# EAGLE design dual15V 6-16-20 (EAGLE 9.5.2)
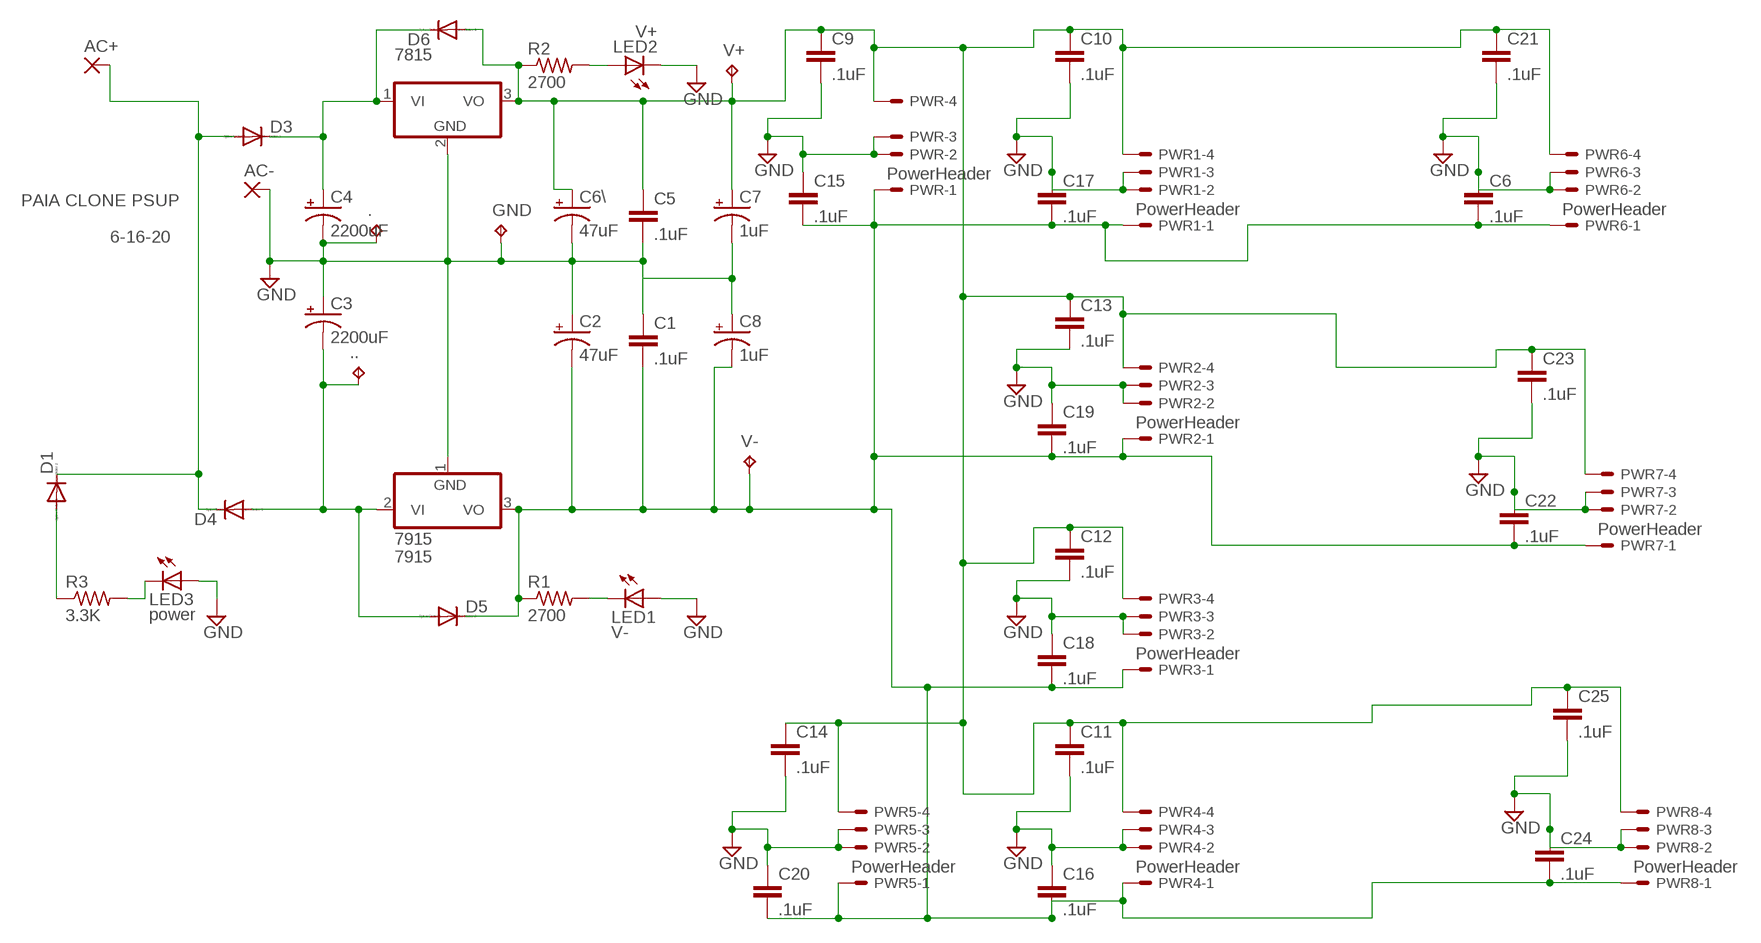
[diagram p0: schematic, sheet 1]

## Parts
7815  7805T  [TO220H]
7915  7915  7905T  [TO220H]
.  TPPAD1-17Y  [P1-17Y]
..  TPPAD1-17Y  [P1-17Y]
AC+  3,17/1,3  [3,17/1,3]
AC-  3,17/1,3  [3,17/1,3]
C1  .1uF  C5/2.5  [C5B2.5]
C2  47uF  CPOL-USE5-8.5  [E5-8,5]
C3  2200uF  CPOL-USE25-10AXIAL  [E25-10]
C4  2200uF  CPOL-USE25-10AXIAL  [E25-10]
C5  .1uF  C5/2.5  [C5B2.5]
C6  .1uF  C2.5/2  [C2.5-2]
C6\  47uF  CPOL-USE5-8.5  [E5-8,5]
C7  1uF  CPOL-USE5-8.5  [E5-8,5]
C8  1uF  CPOL-USE5-8.5  [E5-8,5]
C9  .1uF  C2.5/2  [C2.5-2]
C10  .1uF  C2.5/2  [C2.5-2]
C11  .1uF  C2.5/2  [C2.5-2]
C12  .1uF  C2.5/2  [C2.5-2]
C13  .1uF  C2.5/2  [C2.5-2]
C14  .1uF  C2.5/2  [C2.5-2]
C15  .1uF  C2.5/2  [C2.5-2]
C16  .1uF  C2.5/2  [C2.5-2]
C17  .1uF  C2.5/2  [C2.5-2]
C18  .1uF  C2.5/2  [C2.5-2]
C19  .1uF  C2.5/2  [C2.5-2]
C20  .1uF  C2.5/2  [C2.5-2]
C21  .1uF  C2.5/2  [C2.5-2]
C22  .1uF  C2.5/2  [C2.5-2]
C23  .1uF  C2.5/2  [C2.5-2]
C24  .1uF  C2.5/2  [C2.5-2]
C25  .1uF  C2.5/2  [C2.5-2]
D1  1N4004  [DO41-10]
D3  1N4004  [DO41-10]
D4  1N4004  [DO41-10]
D5  1N4004  [DO41-10]
D6  1N4004  [DO41-10]
GND  TPPAD1-17Y  [P1-17Y]
LED1  V-  LEDB156  [Q62902-B156]
LED2  V+  LEDB156  [Q62902-B156]
LED3  power  LEDB156  [Q62902-B156]
PWR  PowerHeader  C-GRID-04-70543  [70543-04]
PWR1  PowerHeader  C-GRID-04-70543  [70543-04]
PWR2  PowerHeader  C-GRID-04-70543  [70543-04]
PWR3  PowerHeader  C-GRID-04-70543  [70543-04]
PWR4  PowerHeader  C-GRID-04-70543  [70543-04]
PWR5  PowerHeader  C-GRID-04-70543  [70543-04]
PWR6  PowerHeader  C-GRID-04-70543  [70543-04]
PWR7  PowerHeader  C-GRID-04-70543  [70543-04]
PWR8  PowerHeader  C-GRID-04-70543  [70543-04]
R1  2700  R-US_0204/7  [0204/7]
R2  2700  R-US_0204/7  [0204/7]
R3  3.3K  R-US_0204/7  [0204/7]
V+  TPPAD1-17Y  [P1-17Y]
V-  TPPAD1-17Y  [P1-17Y]

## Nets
GND: 7815.2(GND) 7915.1(GND) ..TP AC-.1(P) C1.1 C2.+ C3.+ C4.- C5.2 C6.1 C6\.- C7.- C8.+ C9.2 C10.2 C11.2 C12.2 C13.2 C14.2 C15.1 C16.1 C17.1 C18.1 C19.1 C20.1 C21.2 C22.1 C23.2 C24.1 C25.2 GND.TP LED1.A LED2.K(C) LED3.A PWR1.2 PWR1.3 PWR2.2 PWR2.3 PWR3.2 PWR3.3 PWR4.2 PWR4.3 PWR5.2 PWR5.3 PWR6.2 PWR6.3 PWR7.2 PWR7.3 PWR8.2 PWR8.3 PWR.2 PWR.3
N$1: 7815.1(VI) C4.+ D3.C D6.C
N$2: AC+.1(P) D1.C D3.A D4.C
N$3: LED3.K(C) R3.2
N$4: D1.A R3.1
N$5: LED2.A R2.2
N$6: 7915.2(VI) ...TP C3.- D4.A D5.A
N$7: LED1.K(C) R1.2
V+15: 7815.3(VO) C5.1 C6\.+ C7.+ C9.1 C10.1 C11.1 C12.1 C13.1 C14.1 C21.1 C23.1 C25.1 D6.A PWR1.4 PWR2.4 PWR3.4 PWR4.4 PWR5.4 PWR6.4 PWR7.4 PWR8.4 PWR.4 R2.1 V+.TP
V-15: 7915.3(VO) C1.2 C2.- C6.2 C8.- C15.2 C16.2 C17.2 C18.2 C19.2 C20.2 C22.2 C24.2 D5.C PWR1.1 PWR2.1 PWR3.1 PWR4.1 PWR5.1 PWR6.1 PWR7.1 PWR8.1 PWR.1 R1.1 V-.TP

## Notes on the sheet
- PAIA CLONE PSUP
- 6-16-20

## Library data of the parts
7815 = linear:78*: Positive VOLTAGE REGULATOR Source: http://cache.national.com/ds/LM/LM78L05.pdf http://www.fairchildsemi.com/ds/LM/LM7805.pdf
7915 = linear:79*: Negative VOLTAGE REGULATOR
. .. GND V+ V- = testpad:TP: Test pad
AC+ AC- = wirepad:3,17/1,3: THROUGH-HOLE PAD
C1 C5 C6 C9-C25 = capacitor-wima:C: CAPACITOR
C2-C4 C6\ C7 C8 = rcl:CPOL-US: POLARIZED CAPACITOR, American symbol; SPICEPREFIX: C
D1 D3-D6 = diode:1N4004: DIODE
LED1-LED3 = led:LED: LED
PWR PWR1-PWR8 = con-molex:C-GRID-04: CONNECTOR wire to board 2.54 mm (0.100") pitch header; MF: MOLEX; OC_FARNELL: unknown; OC_NEWARK: unknown
R1-R3 = rcl:R-US_: RESISTOR, American symbol

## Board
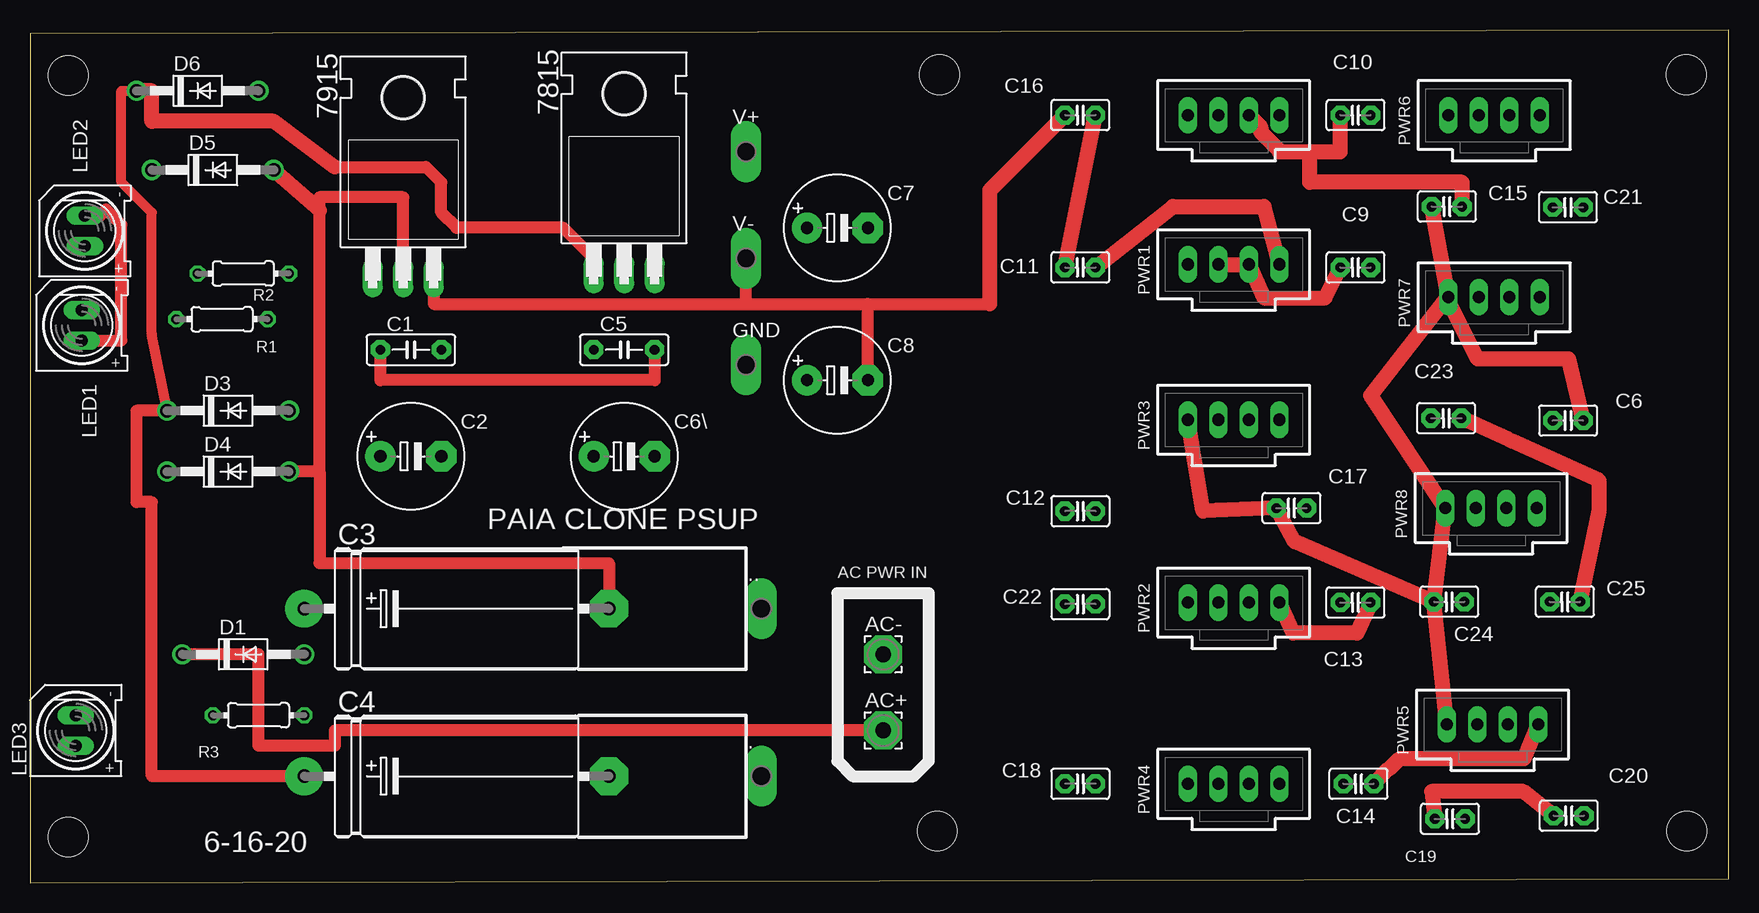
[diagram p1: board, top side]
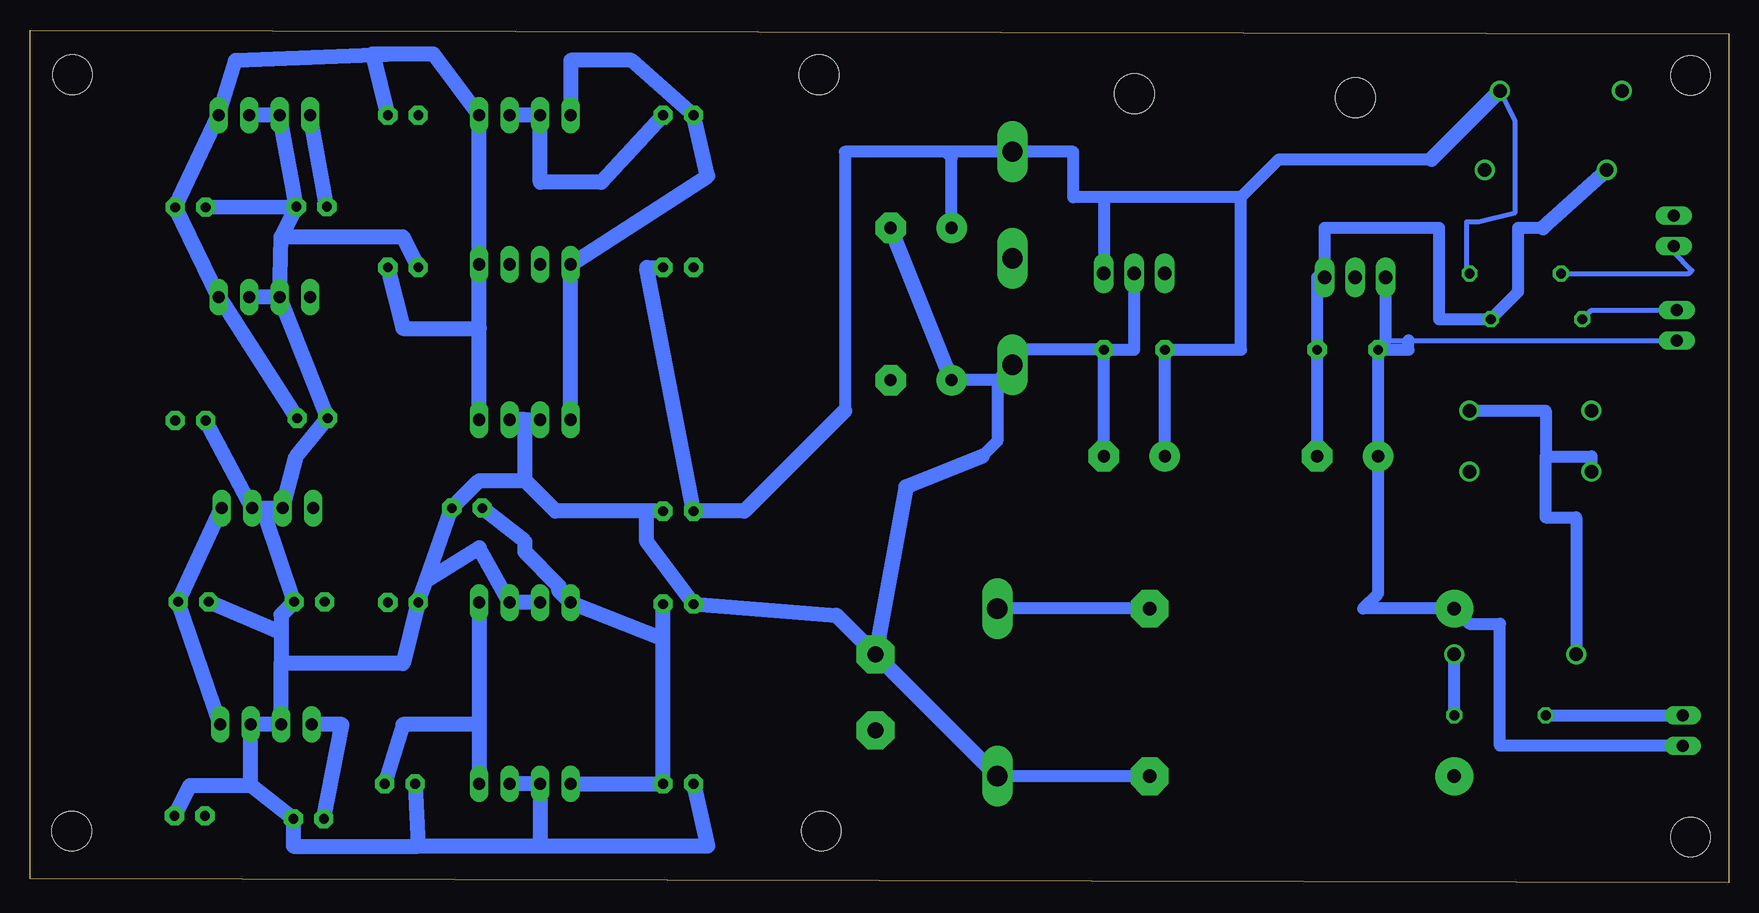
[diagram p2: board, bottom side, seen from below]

Size 141.59 x 71.11 mm. Coordinates in mm from the lower left corner, seen from the top.
Outline: 0,0 141.59,0.32 141.59,71.11 0,70.79 0,0
Copper layers (1*16): Top 0.035mm / dielectric 1.5mm / Bottom 0.035mm
Design rules "default": minimum track width 6mil, minimum drill 0.35mm, track to track 6mil, track to pad 6mil, pad to pad 6mil, via to via 6mil, smd to smd 6mil, copper to edge 40mil, drill to drill 6mil, minimum pad ring 10mil, minimum via ring 8mil, stop-mask expansion 4mil, vias tented up to drill 0mil, thermal gap 10mil
Holes 3.3 mm at 3.17,3.81 75.63,4.32 75.82,67.37 3.17,67.31 138.05,67.37 138.11,4.32

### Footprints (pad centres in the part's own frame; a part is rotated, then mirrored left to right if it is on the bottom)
TO220H = drill 1.118 long: 1 -2.54,-10.16; 2 0,-10.16; 3 2.54,-10.16 | hole 3.302: 0,4.826
P1-17Y = drill 1.702 pad 2.121 long: TP 0,0
3,17/1,3 = drill 1.321 pad 3.175 octagon: 1 0,0
C5B2.5 = drill 0.813 pad 1.6 octagon: 1 -2.54,0; 2 2.54,0
E5-8,5 = drill 1.016 pad 2.54: + -2.54,0 | drill 1.016 pad 2.54 octagon: - 2.54,0
E25-10 = drill 1.118 pad 3.15: + -12.7,0 | drill 1.118 pad 3.15 octagon: - 12.7,0
C2.5-2 = drill 0.813 pad 1.6 octagon: 1 -1.27,0; 2 1.27,0
DO41-10 = drill 1.118: A 5.08,0; C -5.08,0
Q62902-B156 = drill 1.016 long: A -1.27,0; K 1.27,0
70543-04 = drill 1.016 long: 1 -3.81,0; 2 -1.27,0; 3 1.27,0; 4 3.81,0
0204/7 = drill 0.813 octagon: 1 -3.81,0; 2 3.81,0

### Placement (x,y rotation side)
7815  49.53,60.96 0 top
7915  31.11,60.64 0 top
.  60.96,8.89 0 top
..  60.96,22.86 0 top
AC+  71.12,12.7 0 top
AC-  71.12,19.05 0 top
C1  31.75,44.45 0 top
C2  31.75,35.56 0 top
C3  35.56,22.86 0 top
C4  35.56,8.89 0 top
C5  49.53,44.45 0 top
C6  128.21,38.54 0 top
C6\  49.53,35.56 0 top
C7  67.31,54.61 0 top
C8  67.31,41.91 0 top
C9  110.49,51.31 180 top
C10  110.49,64.01 180 top
C11  87.55,51.31 180 top
C12  87.55,30.99 0 top
C13  110.49,23.37 180 top
C14  110.74,8.25 180 top
C15  118.11,56.39 180 top
C16  87.55,64.01 180 top
C17  105.16,31.24 180 top
C18  87.55,8.25 0 top
C19  118.36,5.33 180 top
C20  128.27,5.59 180 top
C21  128.21,56.32 180 top
C22  87.55,23.24 0 top
C23  118.05,38.73 180 top
C24  118.3,23.43 180 top
C25  127.95,23.43 180 top
D1  17.78,19.05 0 top
D3  16.51,39.37 0 top
D4  16.51,34.29 0 top
D5  15.24,59.44 0 top
D6  13.97,66.04 0 top
GND  59.69,43.18 0 top
LED1  4.32,46.48 90 top
LED2  4.57,54.36 90 top
LED3  3.81,12.7 90 top
PWR  100.33,64.01 0 top
PWR1  100.33,51.56 0 top
PWR2  100.33,23.37 0 top
PWR3  100.33,38.61 0 top
PWR4  100.33,8.25 0 top
PWR5  121.92,13.21 0 top
PWR6  122.05,64.01 0 top
PWR7  122.05,48.83 0 top
PWR8  121.79,31.24 0 top
R1  16,46.99 180 top
R2  17.78,50.8 180 top
R3  19.05,13.97 180 top
V+  59.69,60.96 0 top
V-  59.69,52.07 0 top

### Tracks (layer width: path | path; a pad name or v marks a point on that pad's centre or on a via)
GND
  Top 1.016: C5.2 52.07,41.91 29.21,41.91 C1.1 | LED1.A 7.62,45.21 7.62,54.86 6.35,56.13 5.84,55.63 LED2.K
  Top 1.27: C11.2 C16.1 | PWR1.2 PWR1.3 102.87,48.77 107.95,48.77 C9.2 | PWR.3 102.59,63.02 102.59,62.6 104.14,61.06 104.14,60.96 106.68,60.96 | 106.68,60.96 109.22,60.96 C10.2 | C15.1 119.38,58.42 106.68,58.42 106.68,60.96
  Bottom 0.406: 28.57,45.21 26.67,45.21 LED1.A
  Bottom 1.016: C5.2 49.53,44.45 7815.2 | C5.2 59.69,44.45 GND.TP 60.96,41.91 | C6\.- C5.2 | C4.- ..TP | 28.57,45.21 7915.1 | 60.96,41.91 60.96,36.83 62.23,35.56 | 60.96,41.91 C8.+ | LED3.A 19.05,11.43 19.05,21.59 21.59,21.59 C3.+ 30.48,22.86 29.21,24.13 C2.+ C1.1 26.67,44.45 26.67,45.21
  Bottom 1.27: PWR2.2 PWR2.3 104.14,27.94 108.58,25.17 | C12.2 90.17,30.99 | 90.17,30.99 97.79,30.99 100.33,33.53 | 100.33,33.53 100.33,38.61 | 100.33,38.61 PWR3.2 | 100.33,38.61 PWR3.3 | 100.33,33.53 104.14,33.53 C17.1 108.58,25.17 | 90.17,30.99 90.17,28.45 C22.1 74.38,22.31 AC-.1 | 120.65,18.29 110.49,18.29 C13.2 108.58,25.17 | 120.65,20.83 120.65,22.35 C24.1 121.92,30.48 PWR8.3 | 120.65,20.83 120.65,18.29 | 62.23,35.56 68.58,33.02 AC-.1 | ..TP AC-.1 | C15.1 119.74,58.35 PWR6.2 PWR6.3 | PWR7.2 C23.2 119.38,35.56 PWR8.2 PWR8.3 | C18.1 85.09,3.05 99.06,3.05 | 99.06,3.05 109.22,3.05 | 109.22,3.05 119.63,3.05 C19.1 123.19,8.13 | C9.2 110.49,53.85 120.65,53.85 | 120.65,53.85 C15.1 | C21.2 C15.1 | PWR7.2 120.65,53.85 | PWR7.2 PWR7.3 | 120.65,18.29 PWR5.2 PWR5.3 123.19,8.13 | C20.1 128.27,8.13 123.19,8.13 | 120.65,20.83 C25.2 | C8.+ C7.- | C16.1 93.98,58.42 99.06,58.42 PWR.2 PWR.3 | PWR8.3 C6.1 | C14.2 109.22,3.05 | PWR4.3 PWR4.2 99.06,3.05
N$1
  Top 0.813: D3.C 10.16,45.72 10.16,55.88 7.62,58.42 7.62,66.04 D6.C
  Top 1.016: C4.+ 10.16,8.89 10.16,31.75 8.89,31.75 8.89,39.37 D3.C | 7815.1 46.99,52.07 44.45,54.61 35.56,54.61 34.29,55.88 34.29,58.42 33.02,59.69 25.4,59.69
  Top 1.27: 25.4,59.69 20.32,63.5 10.16,63.5 10.16,66.04 D6.C
N$2
  Top 1.016: D1.C 19.05,19.05 19.05,11.43 25.4,11.43 25.4,12.7 AC+.1
  Bottom 1.016: D3.A 15.24,39.37 15.24,35.56 | 15.24,35.56 11.43,35.56 D4.C | 15.24,35.56 15.24,30.48 12.7,30.48 D1.C
N$3
  Bottom 1.016: R3.2 LED3.K
N$4
  Bottom 1.016: R3.1 D1.A
N$5
  Bottom 0.406: R2.2 3.3,50.8 3.05,51.05 4.57,52.58 LED2.A
N$6
  Top 1.016: 7915.2 31.11,57.15 24.13,57.15 24.13,56.07 24.13,34.29 | 24.13,34.29 D4.A | 24.13,34.29 24.13,26.67 48.26,26.67 C3.-
  Top 1.27: D5.A 24.13,56.07
  Bottom 1.016: C3.- ...TP
N$7
  Bottom 0.406: LED1.K 11.43,47.75 R1.2
V+15
  Top 1.27: C11.1 95.25,56.39 102.87,56.39 PWR1.4 | C25.1 130.81,30.99 130.81,33.53 123.53,36.83 123.27,36.94 C23.1 | C13.1 110.61,20.83 105.3,20.83 PWR2.4 | C14.1 113.28,9.53 113.35,9.53 114.19,10.37 124.55,10.37 PWR5.4
  Bottom 0.406: R2.1 21.84,51.05 21.84,55.12 20.83,55.12 17.78,55.88 17.78,63.5 D6.A
  Bottom 1.016: 73.66,39.37 73.66,60.96 65.28,60.96 | C6\.+ C5.1 40.64,44.45 40.64,57.15 | 40.64,57.15 52.07,57.15 | 52.07,57.15 7815.3 | 52.07,57.15 54.61,57.15 54.61,60.96 V+.TP 65.28,60.96 | 24.77,60.33 37.47,60.33 40.64,57.15 | C7.+ 64.77,60.45 65.28,60.96
  Bottom 1.27: 73.66,39.37 82.04,30.99 C12.1 90.17,51.31 C11.1 | PWR2.4 104.14,13.21 | 104.14,13.21 PWR4.4 | 111.76,69.09 107.95,69.09 PWR.4 PWR1.4 104.14,46.23 | 111.76,69.09 113.03,69.09 C10.1 | 104.14,13.21 110.49,13.21 C14.1 | PWR3.4 104.14,46.23 | C9.1 110.49,46.23 104.14,46.23 | C23.1 125.73,48.77 PWR7.4 C21.1 PWR6.4 124.46,68.58 111.76,69.09 | PWR5.4 C25.1 PWR8.4 | 24.77,60.33 D6.A
V-15
  Top 1.016: 7915.3 33.66,48.26 59.69,48.26 | 59.69,48.26 V-.TP | 59.69,48.26 69.85,48.26 | 69.85,48.26 80.01,48.26 | C8.- 69.85,48.26
  Top 1.27: C16.2 80.01,57.74 80.01,48.26 | C15.2 PWR7.1 118.11,48.77 | C6.2 128.27,43.69 120.65,43.69 118.11,48.77 | PWR3.1 97.79,30.99 C17.2 105.41,28.45 C24.2 | PWR5.1 C24.2 | C20.2 124.46,7.62 116.84,7.62 C19.2 | C24.2 PWR8.1 111.76,40.64 118.11,48.77
  Bottom 1.016: C2.- C1.2 34.29,50.48 7915.3 33.66,54.61 24.13,54.61 24.13,46.99 R1.1 17.53,49.28 17.53,54.61 15.47,54.61
  Bottom 1.27: C17.2 100.33,28.45 100.33,27.59 97.51,24.77 97.51,24.36 PWR2.1 88.82,20.32 | PWR3.1 PWR1.1 85.09,58.93 C16.2 91.44,68.58 96.52,68.58 PWR.1 | 88.82,20.32 C18.2 PWR4.1 | 88.82,20.32 C22.2 | C15.2 PWR6.1 | C19.2 115.57,13.21 PWR5.1 | 15.47,54.61 D5.C

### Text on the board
tNames: PAIA CLONE PSUP | AC PWR IN | 6-16-20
